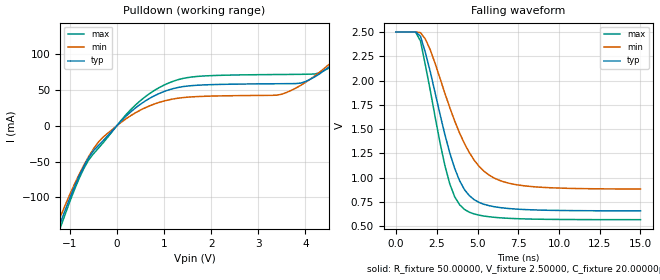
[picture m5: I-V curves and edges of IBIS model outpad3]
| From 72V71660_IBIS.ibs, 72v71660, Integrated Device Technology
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|   Model outpad3
[Model]   outpad3
Model_type   Open_drain
Polarity   Non-Inverting
|Vinl =  0.80000V
|Vinh =  2.00000V
Vmeas =  1.50000V
C_comp   5.00000pF   NA   NA
[Temperature Range]   25.00000   100.00000   0.000
[Voltage Range]   3.30000V   3.00000V   3.60000V
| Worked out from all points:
|   slope of the pulldown table from 0 to 0.495 V, typ, clamps not added: 16.6 ohm
|   falling waveform, R_fixture 50.00000, V_fixture 2.50000, C_fixture 20.00000pF: 20-80 % time 1.72ns typ, 2.3ns min, 1.42ns max; typ from 2.5 V to 0.659 V
[Pulldown]
| voltage   I(typ)   I(min)   I(max)
-3.3V     -522.9mA   -485.5mA   -543.1mA
-1.3V     -153.8mA   -143.1mA   -161.4mA
-1V       -101.9mA   -96.65mA   -106.8mA
-700mV    -56.81mA   -55.31mA   -59.88mA
-400mV    -28.33mA   -23.6mA    -32.16mA
400mV     25.18mA    18.36mA    29.3mA
1.1V      50.23mA    36.28mA    59.89mA
3.5V      58.91mA    44.27mA    71.8mA
4V        61.97mA    60.76mA    72.13mA
4.5V      82.34mA    85.85mA    80.82mA
5.3V      139.5mA    142mA      132.2mA
6.6V      332.3mA    305.7mA    332.7mA
[Ramp]
| variable   typ   min   max
dV/dt_r   1.39320/1.55145n   1.13040/1.90274n   1.59900/1.32996n
dV/dt_f   1.40478/1.61297n   1.10940/2.05411n   1.61436/1.38473n
R_load = 50.00000
[Falling Waveform]
R_fixture = 50.00000
V_fixture = 2.50000
C_fixture = 20.00000pF
R_dut = 129.80000m
L_dut = 9.76000nH
C_dut = 1.23400pF
| time   V(typ)   V(min)   V(max)
0s        2.5V       2.5V       2.5V
1.2ns     2.5V       2.5V       2.498V
1.5ns     2.456V     2.493V     2.407V
2.1ns     2.092V     2.316V     1.899V
3ns       1.443V     1.868V     1.125V
3.6ns     1.096V     1.583V     803.6mV
4.2ns     877.5mV    1.351V     673.9mV
5.4ns     726.6mV    1.067V     605.7mV
6.9ns     683.5mV    944.7mV    582.7mV
15ns      659.1mV    883.7mV    568.4mV
